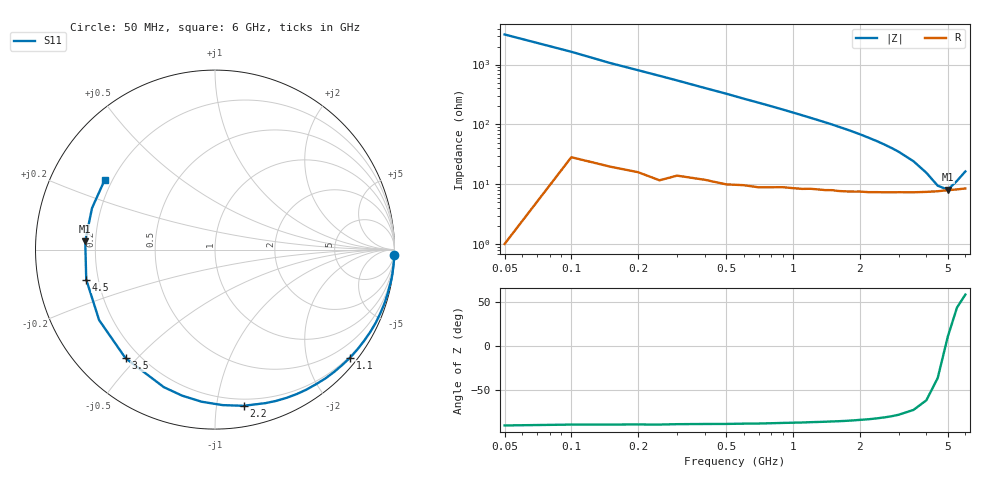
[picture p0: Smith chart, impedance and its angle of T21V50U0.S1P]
! SIEMENS Discrete & RF Semiconductors
! BAS70-04W
! Si Schottky Diode in SOT323
! VR = 1.5 V
! S-Parameters:  November  1997
# GHz  S  MA  R  50
!  f  S11
! GHz  MAG  ANG
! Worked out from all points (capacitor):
!   34 points, 50 MHz to 6 GHz, reference 50 ohm
!   read as one part to ground: C = 1 pF near 50 MHz
!   lowest |Z| = 8.15 ohm at 5 GHz (marker M1)
!   series resonance near 4.89 GHz, so ESL is about 1.1 nH
!   S11 on the Smith chart (normalised r, x): 50 MHz: 0, -64; 1.1 GHz: 0.17, -2.85; 2.2 GHz: 0.15, -1.19; 3.5 GHz: 0.15, -0.46; 4.5 GHz: 0.15, -0.11; 6 GHz: 0.17, +0.28
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0.05  1 -1.8
0.15  0.9982 -5.4
0.25  0.9972 -8.8
0.4  0.9929 -14.0
0.5  0.9909 -17.4
0.6  0.9872 -21.0
0.7  0.9842 -24.4
0.8  0.9794 -27.9
0.9  0.974 -31.4
1.1  0.9638 -38.6
1.3  0.9512 -45.8
1.4  0.9453 -49.4
1.6  0.9319 -56.8
1.7  0.9248 -60.5
1.8  0.9172 -64.2
1.9  0.909 -68.1
2  0.9004 -71.8
2.2  0.8848 -79.6
2.4  0.8675 -87.2
2.6  0.8509 -95.0
2.8  0.8341 -102.7
3  0.8177 -110.4
3.5  0.7838 -129.5
4  0.7557 -148.7
4.5  0.7365 -166.9
5  0.7245 176.3
5.5  0.7231 161.4
6  0.7271 147.7
